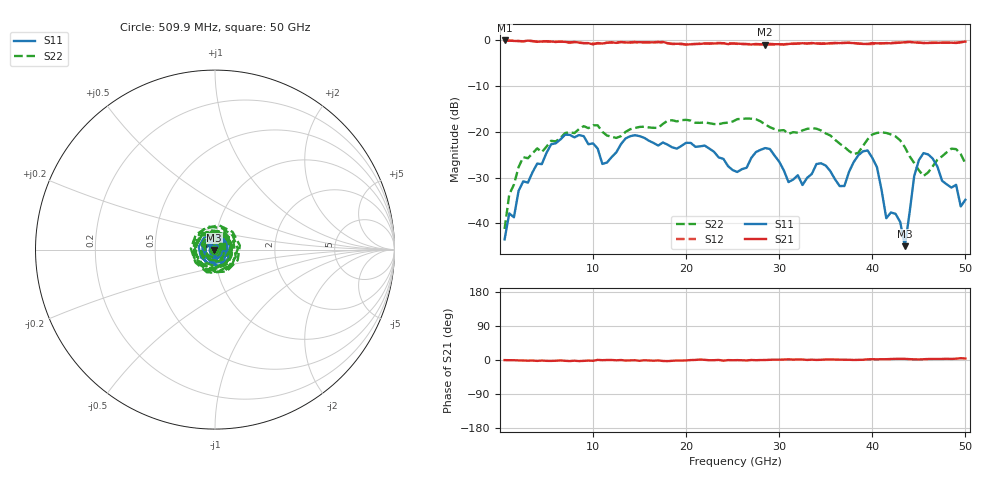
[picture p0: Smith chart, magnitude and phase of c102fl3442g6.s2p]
! 8/2/2019 3:13:32 PM
! Z:\MATT MILLER ENGINEERING\C102FL3442G6.S2P
! CHANNEL.1
! TR.MEASUREMENT
! CORRECTED.DATA
# GHZ S RI R 50.0
! FREQ.GHZ  S11RE  S11IM  S21RE  S21IM  S12RE  S12IM  S22RE  S22IM
!; PortSelection: Port_12
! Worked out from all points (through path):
!   100 points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, 509.9 MHz to 50 GHz, reference 50 ohm
!   highest |S21| = -0.01 dB at 509.9 MHz (marker M1); lowest = -0.9 dB at 28.5 GHz (marker M2)
!   lowest |S11| = -45.0 dB at 43.5 GHz (marker M3), VSWR 1.01, Z = 49.5 - j0.258 ohm
!   |S11| at or under -10 dB: start of sweep to end of sweep
!   |S22| runs from -41.2 to -17.1 dB; largest |S21 - S12| = 0.03
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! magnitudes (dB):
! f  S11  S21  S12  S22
! 509.9 MHz  -43.5  0.0  0.0  -41.2
! 1.01 GHz  -37.8  0.0  -0.1  -33.7
! 2.51 GHz  -30.8  -0.2  -0.2  -25.5
! 5.509 GHz  -22.7  -0.2  -0.3  -21.9
! 9.008 GHz  -20.9  -0.6  -0.6  -18.7
! 11.01 GHz  -27.0  -0.7  -0.7  -20.0
! 14.01 GHz  -20.9  -0.5  -0.4  -19.4
! 17.51 GHz  -22.3  -0.3  -0.5  -18.2
! 25.5 GHz  -28.8  -0.7  -0.8  -17.2
! 28.5 GHz  -23.5  -0.9  -0.9  -18.4
! 31 GHz  -31.0  -0.8  -0.7  -20.4
! 33.5 GHz  -29.2  -0.6  -0.7  -19.2
! 37 GHz  -31.8  -0.5  -0.6  -23.3
! 39.5 GHz  -24.0  -0.8  -0.8  -21.6
! 40.5 GHz  -27.7  -0.6  -0.7  -20.2
! 41.5 GHz  -38.9  -0.6  -0.6  -20.2
! 42 GHz  -37.6  -0.6  -0.5  -20.5
! 43.5 GHz  -45.0  -0.4  -0.4  -23.3
! 44.5 GHz  -29.7  -0.4  -0.4  -26.8
! 45.5 GHz  -24.6  -0.6  -0.6  -29.6
! 48.5 GHz  -32.2  -0.5  -0.5  -23.6
! 50 GHz  -34.8  -0.2  -0.3  -26.9
